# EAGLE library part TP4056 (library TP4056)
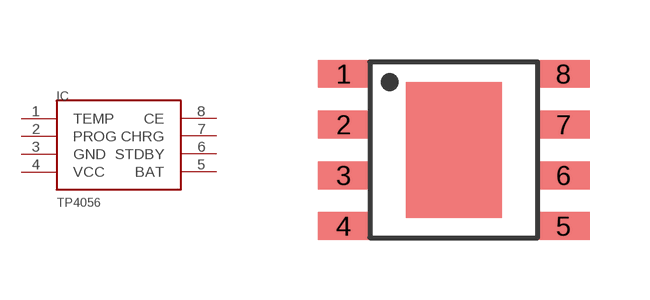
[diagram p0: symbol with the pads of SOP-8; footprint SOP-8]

Designator prefix IC

## TP4056  [SOP-8]
1  TEMP
2  PROG
3  GND
4  VCC
5  BAT
6  STDBY
7  CHRG
8  CE

## Footprint SOP-8 (pad centres in mm)
smd 1.3 x 0.7: 1 -2.75,1.905; 2 -2.75,0.635; 3 -2.75,-0.635; 4 -2.75,-1.905; 5 2.75,-1.905; 6 2.75,-0.635; 7 2.75,0.635; 8 2.75,1.905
